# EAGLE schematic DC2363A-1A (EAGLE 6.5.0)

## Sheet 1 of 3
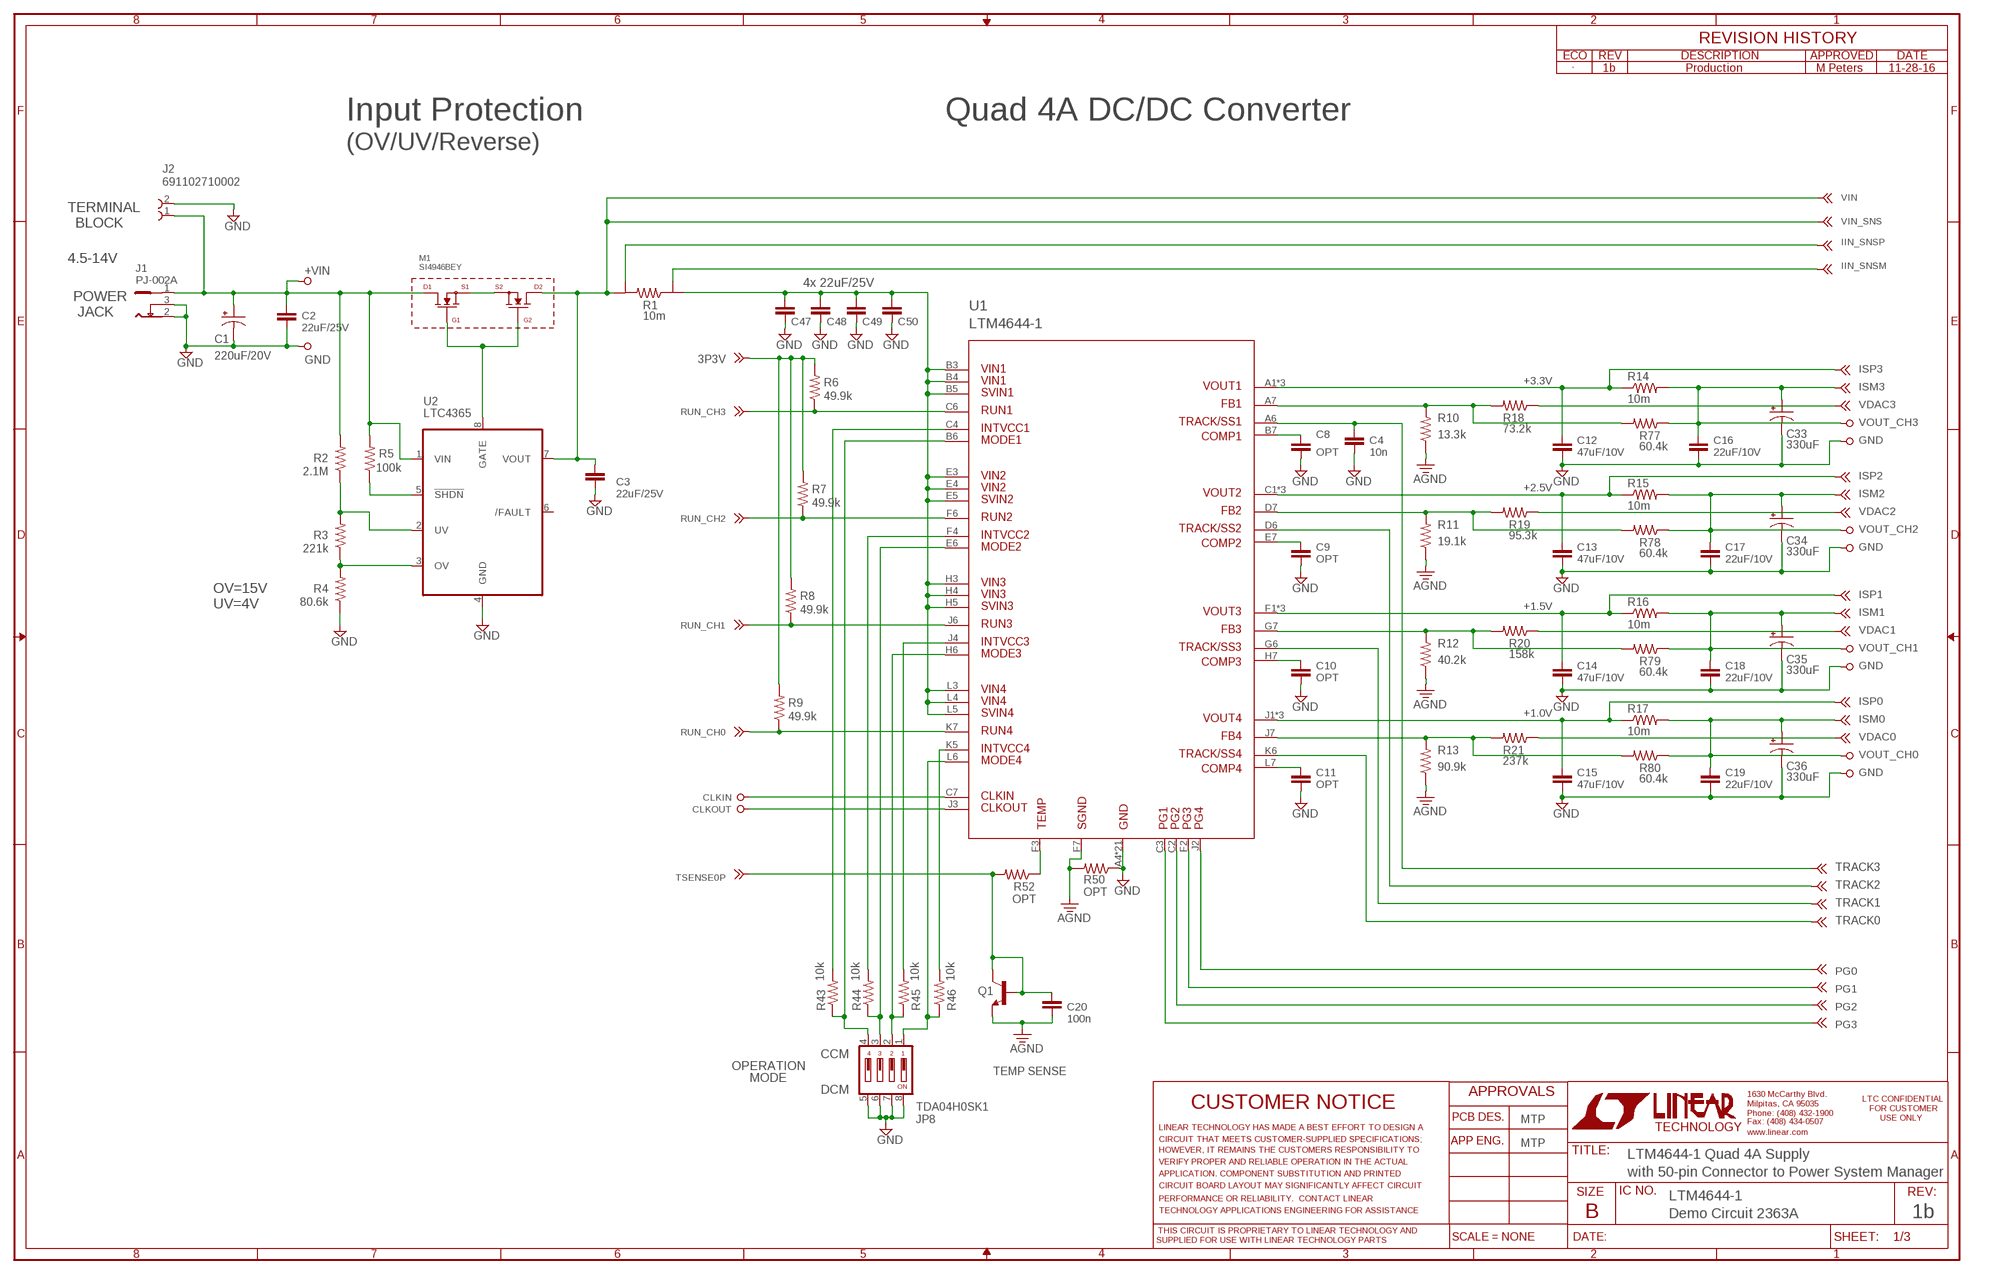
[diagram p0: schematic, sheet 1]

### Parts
C1  220uF/20V  CPOL-USE3.5-8  [E3,5-8]
C2  22uF/25V  CC1210_BOX  [C1210_BOX]
C3  22uF/25V  CC1210_BOX  [C1210_BOX]
C4  10n  CC0603_BOX  [C0603_BOX]
C8  OPT  CC0603_BOX  [C0603_BOX]
C9  OPT  CC0603_BOX  [C0603_BOX]
C10  OPT  CC0603_BOX  [C0603_BOX]
C11  OPT  CC0603_BOX  [C0603_BOX]
C12  47uF/10V  CC1206_BOX  [C1206_BOX]
C13  47uF/10V  CC1206_BOX  [C1206_BOX]
C14  47uF/10V  CC1206_BOX  [C1206_BOX]
C15  47uF/10V  CC1206_BOX  [C1206_BOX]
C16  22uF/10V  CC1210_BOX  [C1210_BOX]
C17  22uF/10V  CC1210_BOX  [C1210_BOX]
C18  22uF/10V  CC1210_BOX  [C1210_BOX]
C19  22uF/10V  CC1210_BOX  [C1210_BOX]
C20  100n  CC0603_BOX  [C0603_BOX]
C33  330uF  CPOL-USD/7343-31R  [D/7343-31R]
C34  330uF  CPOL-USD/7343-31R  [D/7343-31R]
C35  330uF  CPOL-USD/7343-31R  [D/7343-31R]
C36  330uF  CPOL-USD/7343-31R  [D/7343-31R]
C47  22uF/25V  CC1210_BOX  [C1210_BOX]
C48  22uF/25V  CC1210_BOX  [C1210_BOX]
C49  22uF/25V  CC1206_BOX  [C1206_BOX]
C50  22uF/25V  CC1206_BOX  [C1206_BOX]
J1  PJ-002A  [PJ-002A]
J2  691102710002  [691102710002]
JP8  TDA04H0SK1  [SMT_DIP_4]
M1  SI4946BEY  [SOIC-8]
Q1  TEMP SENSE  NPN-SOT23  [SOT-23]
R1  10m  SHUNT  [2512_SHUNT_5MOHM]
R2  2.1M  RR0603_BOX  [R0603_BOX]
R3  221k  RR0603_BOX  [R0603_BOX]
R4  80.6k  RR0603_BOX  [R0603_BOX]
R5  100k  RR0603_BOX  [R0603_BOX]
R6  49.9k  RR0603_BOX  [R0603_BOX]
R7  49.9k  RR0603_BOX  [R0603_BOX]
R8  49.9k  RR0603_BOX  [R0603_BOX]
R9  49.9k  RR0603_BOX  [R0603_BOX]
R10  13.3k  RR0603_BOX  [R0603_BOX]
R11  19.1k  RR0603_BOX  [R0603_BOX]
R12  40.2k  RR0603_BOX  [R0603_BOX]
R13  90.9k  RR0603_BOX  [R0603_BOX]
R14  10m  RR1210_BOX  [R1210_BOX]
R15  10m  RR1210_BOX  [R1210_BOX]
R16  10m  RR1210_BOX  [R1210_BOX]
R17  10m  RR1210_BOX  [R1210_BOX]
R18  73.2k  RR0603_BOX  [R0603_BOX]
R19  95.3k  RR0603_BOX  [R0603_BOX]
R20  158k  RR0603_BOX  [R0603_BOX]
R21  237k  RR0603_BOX  [R0603_BOX]
R43  10k  RR0603_BOX  [R0603_BOX]
R44  10k  RR0603_BOX  [R0603_BOX]
R45  10k  RR0603_BOX  [R0603_BOX]
R46  10k  RR0603_BOX  [R0603_BOX]
R50  OPT  RR0603_BOX  [R0603_BOX]
R52  OPT  RR0603_BOX  [R0603_BOX]
R77  60.4k  RR0603_BOX  [R0603_BOX]
R78  60.4k  RR0603_BOX  [R0603_BOX]
R79  60.4k  RR0603_BOX  [R0603_BOX]
R80  60.4k  RR0603_BOX  [R0603_BOX]
TP1  TURRET_LARGE_2501  [TURRET_LARGE_2501]
TP2  TURRET_LARGE_2501  [TURRET_LARGE_2501]
TP3  TURRET_LARGE_2501  [TURRET_LARGE_2501]
TP4  TURRET_LARGE_2501  [TURRET_LARGE_2501]
TP5  TURRET_LARGE_2501  [TURRET_LARGE_2501]
TP6  TURRET_LARGE_2501  [TURRET_LARGE_2501]
TP7  TURRET_LARGE_2501  [TURRET_LARGE_2501]
TP8  TURRET_LARGE_2501  [TURRET_LARGE_2501]
TP9  TURRET_LARGE_2501  [TURRET_LARGE_2501]
TP10  TURRET_LARGE_2501  [TURRET_LARGE_2501]
TP11  TURRET_SMALL_2308TP  [TURRET_SMALL_2308]
TP12  TURRET_SMALL_2308TP  [TURRET_SMALL_2308]
TP14  TESTPOINT_SMDVIA  [VIA]
TP15  TESTPOINT_SMDVIA  [VIA]
TP16  TESTPOINT_SMDVIA  [VIA]
U1  LTM4644-1  [BGA77_1.27]
U2  LTC4365  [TSOT-23-8]

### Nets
3P3V: R6.2 R7.2 R8.2 R9.2 ; also sheet 3
+VIN: C1.+ C2.1 J1.1 J2.1 M1.7(D1) M1.8(D1) R2.2 R5.2 TP1.TP U2.1(VIN)
AGND: C20.2 Q1.2(E) R10.1 R11.1 R12.1 R13.1 R50.2 U1.F7(SGND)
CLKIN: TP11.TP1 U1.C7(CLKIN)
CLKOUT: TP12.TP1 U1.J3(CLKOUT)
GND: C1.- C2.2 C3.2 C4.2 C8.2 C9.2 C10.2 C11.2 C12.2 C13.2 C14.2 C15.2 C16.2 C17.2 C18.2 C19.2 C33.- C34.- C35.- C36.- C47.2 C48.2 C49.2 C50.2 J1.2 J1.3 J2.2 JP8.5 JP8.6 JP8.7 JP8.8 R4.1 R50.1 TP2.TP TP4.TP TP6.TP TP8.TP TP10.TP U1.A4(GND) U1.A5(GND) U1.B1(GND) U1.B2(GND) U1.C5(GND) U1.D3(GND) U1.D4(GND) U1.D5(GND) U1.E1(GND) U1.E2(GND) U1.F5(GND) U1.G3(GND) U1.G4(GND) U1.G5(GND) U1.H1(GND) U1.H2(GND) U1.J5(GND) U1.K3(GND) U1.K4(GND) U1.L1(GND) U1.L2(GND) U2.4(GND) ; also sheet 2,3
IIN_SNSM: R1.E1 ; also sheet 2
IIN_SNSP: R1.E2 ; also sheet 2
INT1: R43.2 U1.C4(INTVCC1) ; also sheet 2
INT2: R44.2 U1.F4(INTVCC2) ; also sheet 2
INT3: R45.2 U1.J4(INTVCC3) ; also sheet 2
INT4: R46.2 U1.K5(INTVCC4) ; also sheet 2
ISM0: C19.1 C36.+ R17.2 R80.1 TP9.TP ; also sheet 2,3
ISM1: C18.1 C35.+ R16.2 R79.1 TP7.TP ; also sheet 2,3
ISM2: C17.1 C34.+ R15.2 R78.1 TP5.TP ; also sheet 2,3
ISM3: C16.1 C33.+ R14.2 R77.1 TP3.TP ; also sheet 2,3
ISP0: C15.1 R17.1 U1.J1(VOUT4) U1.K1(VOUT4) U1.K2(VOUT4) ; also sheet 2
ISP1: C14.1 R16.1 U1.F1(VOUT3) U1.G1(VOUT3) U1.G2(VOUT3) ; also sheet 2
ISP2: C13.1 R15.1 U1.C1(VOUT2) U1.D1(VOUT2) U1.D2(VOUT2) ; also sheet 2
ISP3: C12.1 R14.1 U1.A1(VOUT1) U1.A2(VOUT1) U1.A3(VOUT1) ; also sheet 2
N$1: M1.2(G1) M1.4(G2) U2.8(GATE)
N$2: M1.1(S1) M1.3(S2)
N$5: R5.1 U2.5(!SHDN)
N$6: R2.1 R3.2 U2.2(UV)
N$7: R3.1 R4.2 U2.3(OV)
N$9: C11.1 U1.L7(COMP4) ; also sheet 3
N$10: C10.1 U1.H7(COMP3) ; also sheet 3
N$11: C9.1 U1.E7(COMP2) ; also sheet 3
N$12: C8.1 U1.B7(COMP1) ; also sheet 3
N$17: R10.2 R18.2 R77.2 U1.A7(FB1) ; also sheet 3
N$18: R11.2 R19.2 R78.2 U1.D7(FB2) ; also sheet 3
N$19: R12.2 R20.2 R79.2 U1.G7(FB3) ; also sheet 3
N$20: R13.2 R21.2 R80.2 U1.J7(FB4) ; also sheet 3
N$42: JP8.1 R46.1 U1.L6(MODE4)
N$43: JP8.2 R45.1 U1.H6(MODE3)
N$52: JP8.3 R44.1 U1.E6(MODE2)
N$53: JP8.4 R43.1 U1.B6(MODE1)
N$58: R52.1 U1.F3(TEMP)
PG0: U1.J2(PG4) ; also sheet 2
PG1: U1.F2(PG3) ; also sheet 2
PG2: U1.C2(PG2) ; also sheet 2
PG3: U1.C3(PG1) ; also sheet 2
RUN_CH0: R9.1 U1.K7(RUN4) ; also sheet 2,3
RUN_CH1: R8.1 U1.J6(RUN3) ; also sheet 2,3
RUN_CH2: R7.1 U1.F6(RUN2) ; also sheet 2,3
RUN_CH3: R6.1 U1.C6(RUN1) ; also sheet 2,3
TRACK0: TP16.1 U1.K6(TRACK4) ; also sheet 3
TRACK1: TP15.1 U1.G6(TRACK3) ; also sheet 3
TRACK2: TP14.1 U1.D6(TRACK2) ; also sheet 3
TRACK3: C4.1 U1.A6(TRACK1) ; also sheet 3
TSENSE0P: C20.1 Q1.1(B) Q1.3(C) R52.2 ; also sheet 2
VDAC0: R21.1 ; also sheet 2
VDAC1: R20.1 ; also sheet 2
VDAC2: R19.1 ; also sheet 2
VDAC3: R18.1 ; also sheet 2
VIN: C3.1 M1.5(D2) M1.6(D2) R1.I2 U2.7(VOUT) ; also sheet 2,3
VIN_U1: C47.1 C48.1 C49.1 C50.1 R1.I1 U1.B3(VIN1) U1.B4(VIN1) U1.B5(SVIN1) U1.E3(VIN2) U1.E4(VIN2) U1.E5(SVIN2) U1.H3(VIN3) U1.H4(VIN3) U1.H5(SVIN3) U1.L3(VIN4) U1.L4(VIN4) U1.L5(SVIN4)
Unconnected: U2.6(/FAULT)

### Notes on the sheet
- 1b | Production | M Peters | 11-28-16
- Input Protection | Quad 4A DC/DC Converter
- (OV/UV/Reverse)
- VIN_SNS
- TERMINAL
    BLOCK
- 4.5-14V
- +VIN
- 4x 22uF/25V
- POWER
   JACK
- GND
- +3.3V
- VOUT_CH3
- +2.5V
- VOUT_CH2
- OV=15V
  UV=4V
- +1.5V
- VOUT_CH1
- +1.0V
- VOUT_CH0
- CCM
- OPERATION
- MODE
- DCM
- MTP
- MTP
- LTM4644-1 Quad 4A Supply
- with 50-pin Connector to Power System Manager
- LTM4644-1
- Demo Circuit 2363A | 1b

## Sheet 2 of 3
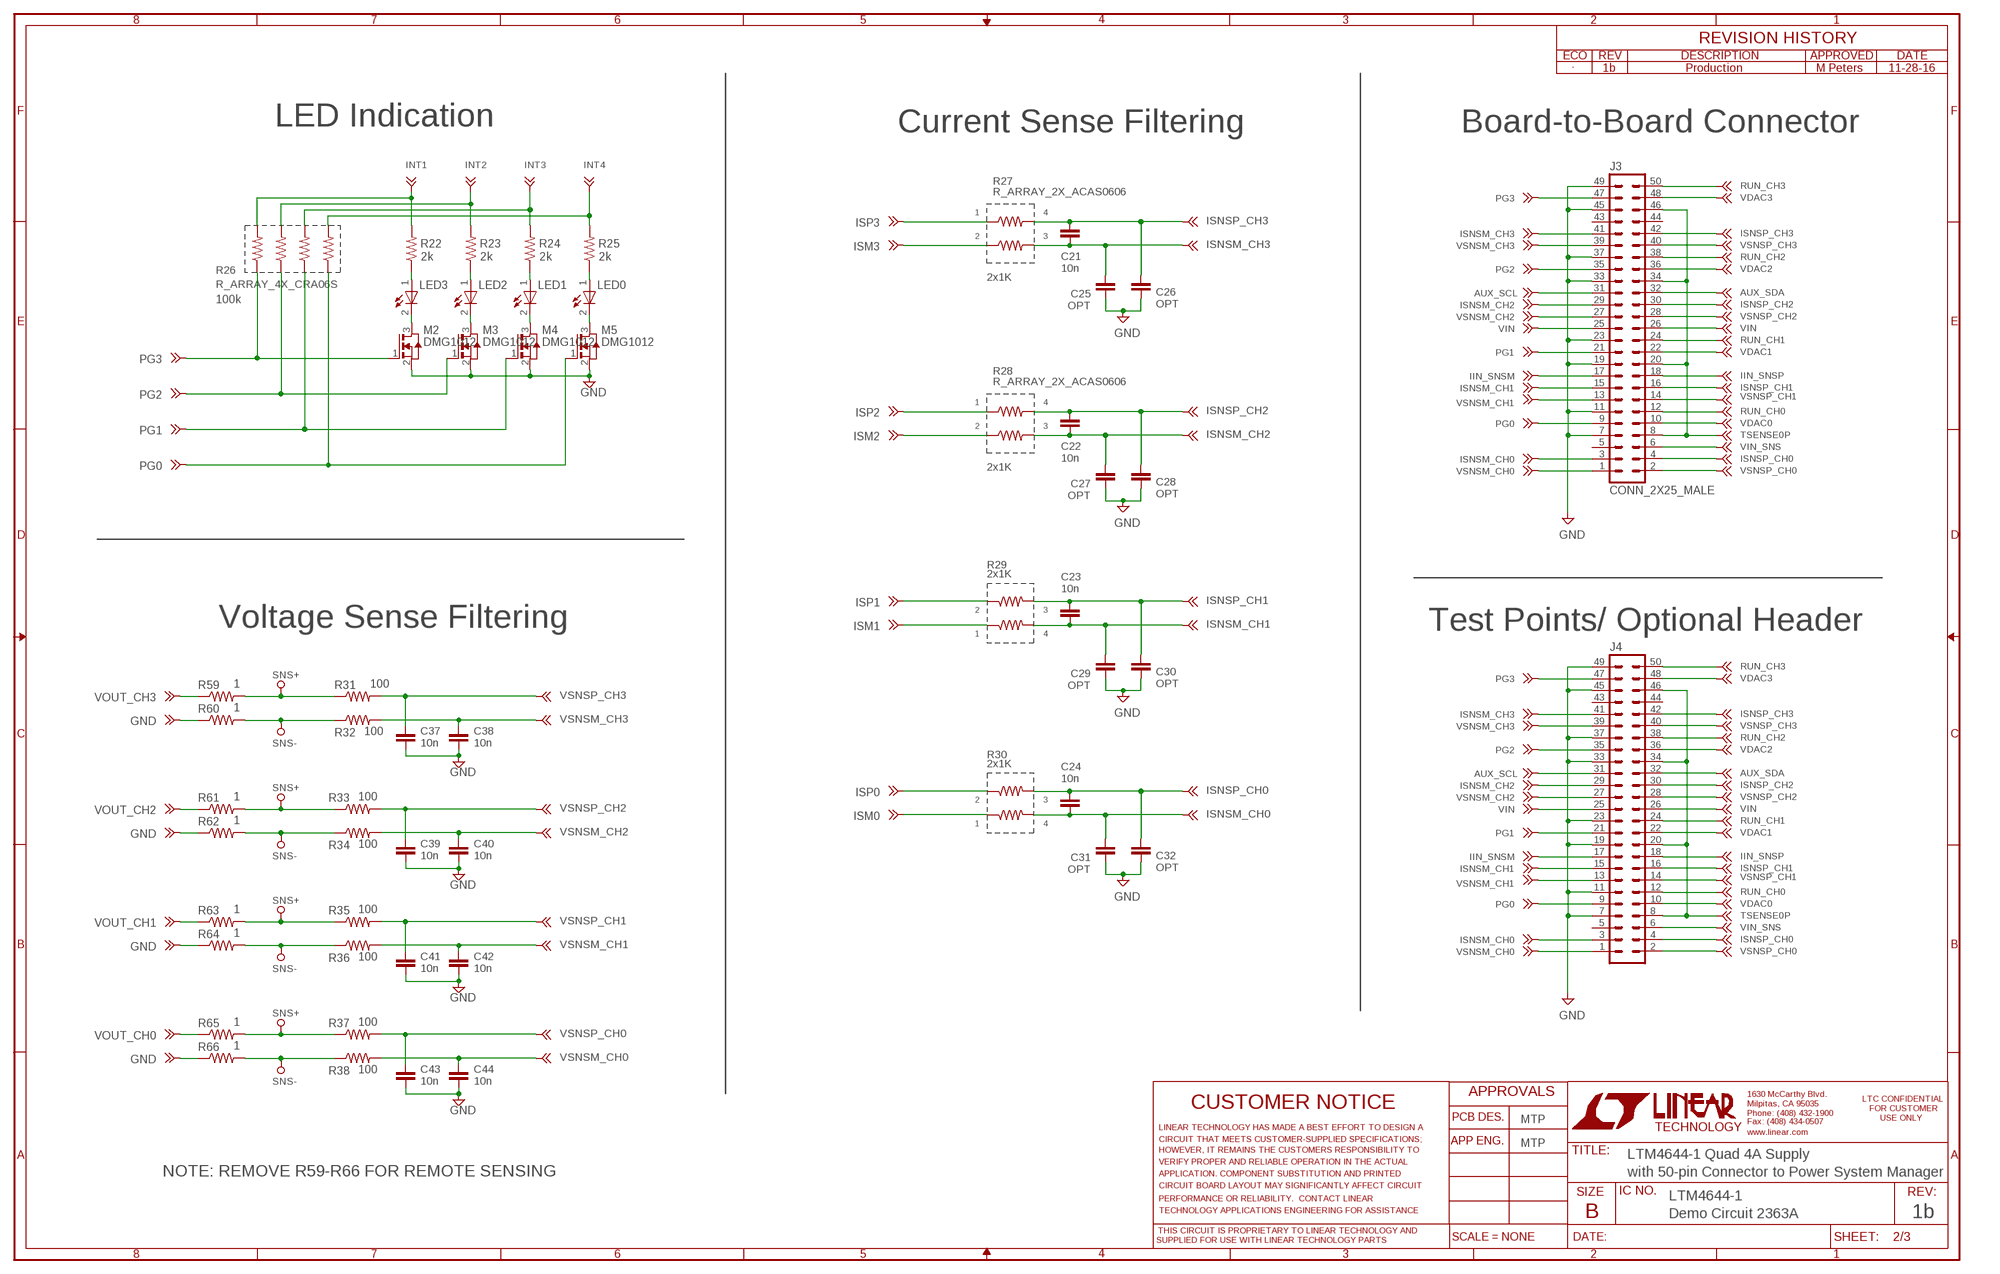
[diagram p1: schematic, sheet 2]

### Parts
C21  10n  CC0603_BOX  [C0603_BOX]
C22  10n  CC0603_BOX  [C0603_BOX]
C23  10n  CC0603_BOX  [C0603_BOX]
C24  10n  CC0603_BOX  [C0603_BOX]
C25  OPT  CC0603_BOX  [C0603_BOX]
C26  OPT  CC0603_BOX  [C0603_BOX]
C27  OPT  CC0603_BOX  [C0603_BOX]
C28  OPT  CC0603_BOX  [C0603_BOX]
C29  OPT  CC0603_BOX  [C0603_BOX]
C30  OPT  CC0603_BOX  [C0603_BOX]
C31  OPT  CC0603_BOX  [C0603_BOX]
C32  OPT  CC0603_BOX  [C0603_BOX]
C37  10n  CC0603_BOX  [C0603_BOX]
C38  10n  CC0603_BOX  [C0603_BOX]
C39  10n  CC0603_BOX  [C0603_BOX]
C40  10n  CC0603_BOX  [C0603_BOX]
C41  10n  CC0603_BOX  [C0603_BOX]
C42  10n  CC0603_BOX  [C0603_BOX]
C43  10n  CC0603_BOX  [C0603_BOX]
C44  10n  CC0603_BOX  [C0603_BOX]
J3  CONN_2X25_MALE  [PINHEAD_2X25_MALE]
J4  CONN_2X25_MALE_NO_SILK  [PINHEAD_2X25_MALE_NO_SILK]
LED0  LED-0603  [CHIPLED_0603]
LED1  LED-0603  [CHIPLED_0603]
LED2  LED-0603  [CHIPLED_0603]
LED3  LED-0603  [CHIPLED_0603]
M2  DMG1012  [SOT-323]
M3  DMG1012  [SOT-323]
M4  DMG1012  [SOT-323]
M5  DMG1012  [SOT-323]
R22  2k  RR0603_BOX  [R0603_BOX]
R23  2k  RR0603_BOX  [R0603_BOX]
R24  2k  RR0603_BOX  [R0603_BOX]
R25  2k  RR0603_BOX  [R0603_BOX]
R26  R_ARRAY_4X_CRA06S  [R_VISHAY_CRA06S]
R27  R_ARRAY_2X_ACAS0606  [R_ARRAY_2X_ACAS]
R28  R_ARRAY_2X_ACAS0606  [R_ARRAY_2X_ACAS]
R29  R_ARRAY_2X_ACAS0606  [R_ARRAY_2X_ACAS]
R30  R_ARRAY_2X_ACAS0606  [R_ARRAY_2X_ACAS]
R31  100  RR0603_BOX  [R0603_BOX]
R32  100  RR0603_BOX  [R0603_BOX]
R33  100  RR0603_BOX  [R0603_BOX]
R34  100  RR0603_BOX  [R0603_BOX]
R35  100  RR0603_BOX  [R0603_BOX]
R36  100  RR0603_BOX  [R0603_BOX]
R37  100  RR0603_BOX  [R0603_BOX]
R38  100  RR0603_BOX  [R0603_BOX]
R59  1  RR0603_BOX  [R0603_BOX]
R60  1  RR0603_BOX  [R0603_BOX]
R61  1  RR0603_BOX  [R0603_BOX]
R62  1  RR0603_BOX  [R0603_BOX]
R63  1  RR0603_BOX  [R0603_BOX]
R64  1  RR0603_BOX  [R0603_BOX]
R65  1  RR0603_BOX  [R0603_BOX]
R66  1  RR0603_BOX  [R0603_BOX]
TP17  TURRET_SMALL_2308TP  [TURRET_SMALL_2308]
TP18  TURRET_SMALL_2308TP  [TURRET_SMALL_2308]
TP19  TURRET_SMALL_2308TP  [TURRET_SMALL_2308]
TP20  TURRET_SMALL_2308TP  [TURRET_SMALL_2308]
TP21  TURRET_SMALL_2308TP  [TURRET_SMALL_2308]
TP22  TURRET_SMALL_2308TP  [TURRET_SMALL_2308]
TP23  TURRET_SMALL_2308TP  [TURRET_SMALL_2308]
TP24  TURRET_SMALL_2308TP  [TURRET_SMALL_2308]

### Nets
AUX_SCL: J3.31 J4.31 ; also sheet 3
AUX_SDA: J3.32 J4.32 ; also sheet 3
GND: C25.1 C26.1 C27.1 C28.1 C29.1 C30.1 C31.1 C32.1 C37.2 C38.2 C39.2 C40.2 C41.2 C42.2 C43.2 C44.2 J3.7 J3.11 J3.19 J3.23 J3.33 J3.37 J3.45 J3.49 J4.7 J4.11 J4.19 J4.23 J4.33 J4.37 J4.45 J4.49 M2.2(S) M3.2(S) M4.2(S) M5.2(S) R60.1 R62.1 R64.1 R66.1 ; also sheet 1,3
IIN_SNSM: J3.17 J4.17 ; also sheet 1
IIN_SNSP: J3.18 J4.18 ; also sheet 1
INT1: R22.2 R26.R1_2 ; also sheet 1
INT2: R23.2 R26.R2_2 ; also sheet 1
INT3: R24.2 R26.R3_2 ; also sheet 1
INT4: R25.2 R26.R4_2 ; also sheet 1
ISM0: R30.P$1 R65.1 ; also sheet 1,3
ISM1: R29.P$1 R63.1 ; also sheet 1,3
ISM2: R28.P$2 R61.1 ; also sheet 1,3
ISM3: R27.P$2 R59.1 ; also sheet 1,3
ISNSM_CH0: C24.2 C31.2 J3.3 J4.3 R30.P$4
ISNSM_CH1: C23.2 C29.2 J3.15 J4.15 R29.P$4
ISNSM_CH2: C22.2 C27.2 J3.29 J4.29 R28.P$3
ISNSM_CH3: C21.2 C25.2 J3.41 J4.41 R27.P$3
ISNSP_CH0: C24.1 C32.2 J3.4 J4.4 R30.P$3
ISNSP_CH1: C23.1 C30.2 J3.16 J4.16 R29.P$3
ISNSP_CH2: C22.1 C28.2 J3.30 J4.30 R28.P$4
ISNSP_CH3: C21.1 C26.2 J3.42 J4.42 R27.P$4
ISP0: R30.P$2 ; also sheet 1
ISP1: R29.P$2 ; also sheet 1
ISP2: R28.P$1 ; also sheet 1
ISP3: R27.P$1 ; also sheet 1
N$27: LED3.P(A) R22.1
N$28: LED2.P(A) R23.1
N$30: LED1.P(A) R24.1
N$31: LED0.P(A) R25.1
N$32: LED3.N(C) M2.3(D)
N$33: LED2.N(C) M3.3(D)
N$34: R31.1 R59.2 TP17.TP1
N$35: R32.1 R60.2 TP18.TP1
N$38: R33.1 R61.2 TP19.TP1
N$39: R34.1 R62.2 TP20.TP1
N$40: LED1.N(C) M4.3(D)
N$41: LED0.N(C) M5.3(D)
N$44: R35.1 R63.2 TP21.TP1
N$45: R36.1 R64.2 TP22.TP1
N$48: R37.1 R65.2 TP23.TP1
N$49: R38.1 R66.2 TP24.TP1
PG0: J3.9 J4.9 M5.1(G) R26.R4_1 ; also sheet 1
PG1: J3.21 J4.21 M4.1(G) R26.R3_1 ; also sheet 1
PG2: J3.35 J4.35 M3.1(G) R26.R2_1 ; also sheet 1
PG3: J3.47 J4.47 M2.1(G) R26.R1_1 ; also sheet 1
RUN_CH0: J3.12 J4.12 ; also sheet 1,3
RUN_CH1: J3.24 J4.24 ; also sheet 1,3
RUN_CH2: J3.38 J4.38 ; also sheet 1,3
RUN_CH3: J3.50 J4.50 ; also sheet 1,3
TSENSE0P: J3.8 J3.20 J3.34 J3.46 J4.8 J4.20 J4.34 J4.46 ; also sheet 1
VDAC0: J3.10 J4.10 ; also sheet 1
VDAC1: J3.22 J4.22 ; also sheet 1
VDAC2: J3.36 J4.36 ; also sheet 1
VDAC3: J3.48 J4.48 ; also sheet 1
VIN: J3.6 J3.25 J3.26 J4.6 J4.25 J4.26 ; also sheet 1,3
VSNSM_CH0: C44.1 J3.1 J4.1 R38.2
VSNSM_CH1: C42.1 J3.13 J4.13 R36.2
VSNSM_CH2: C40.1 J3.27 J4.27 R34.2
VSNSM_CH3: C38.1 J3.39 J4.39 R32.2
VSNSP_CH0: C43.1 J3.2 J4.2 R37.2
VSNSP_CH1: C41.1 J3.14 J4.14 R35.2
VSNSP_CH2: C39.1 J3.28 J4.28 R33.2
VSNSP_CH3: C37.1 J3.40 J4.40 R31.2
Unconnected: J3.5 J3.43 J3.44 J4.5 J4.43 J4.44

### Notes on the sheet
- 1b | Production | M Peters | 11-28-16
- LED Indication | Current Sense Filtering | Board-to-Board Connector
- 2x1K
- 100k
- VIN_SNS
- 2x1K
- 2x1K
- Voltage Sense Filtering | Test Points/ Optional Header
- SNS+
- VOUT_CH3
- SNS-
- 2x1K
- SNS+
- VOUT_CH2
- SNS-
- SNS+
- VOUT_CH1
- VIN_SNS
- SNS-
- SNS+
- VOUT_CH0
- SNS-
- MTP
- MTP
- LTM4644-1 Quad 4A Supply
- NOTE: REMOVE R59-R66 FOR REMOTE SENSING | with 50-pin Connector to Power System Manager
- LTM4644-1
- Demo Circuit 2363A | 1b

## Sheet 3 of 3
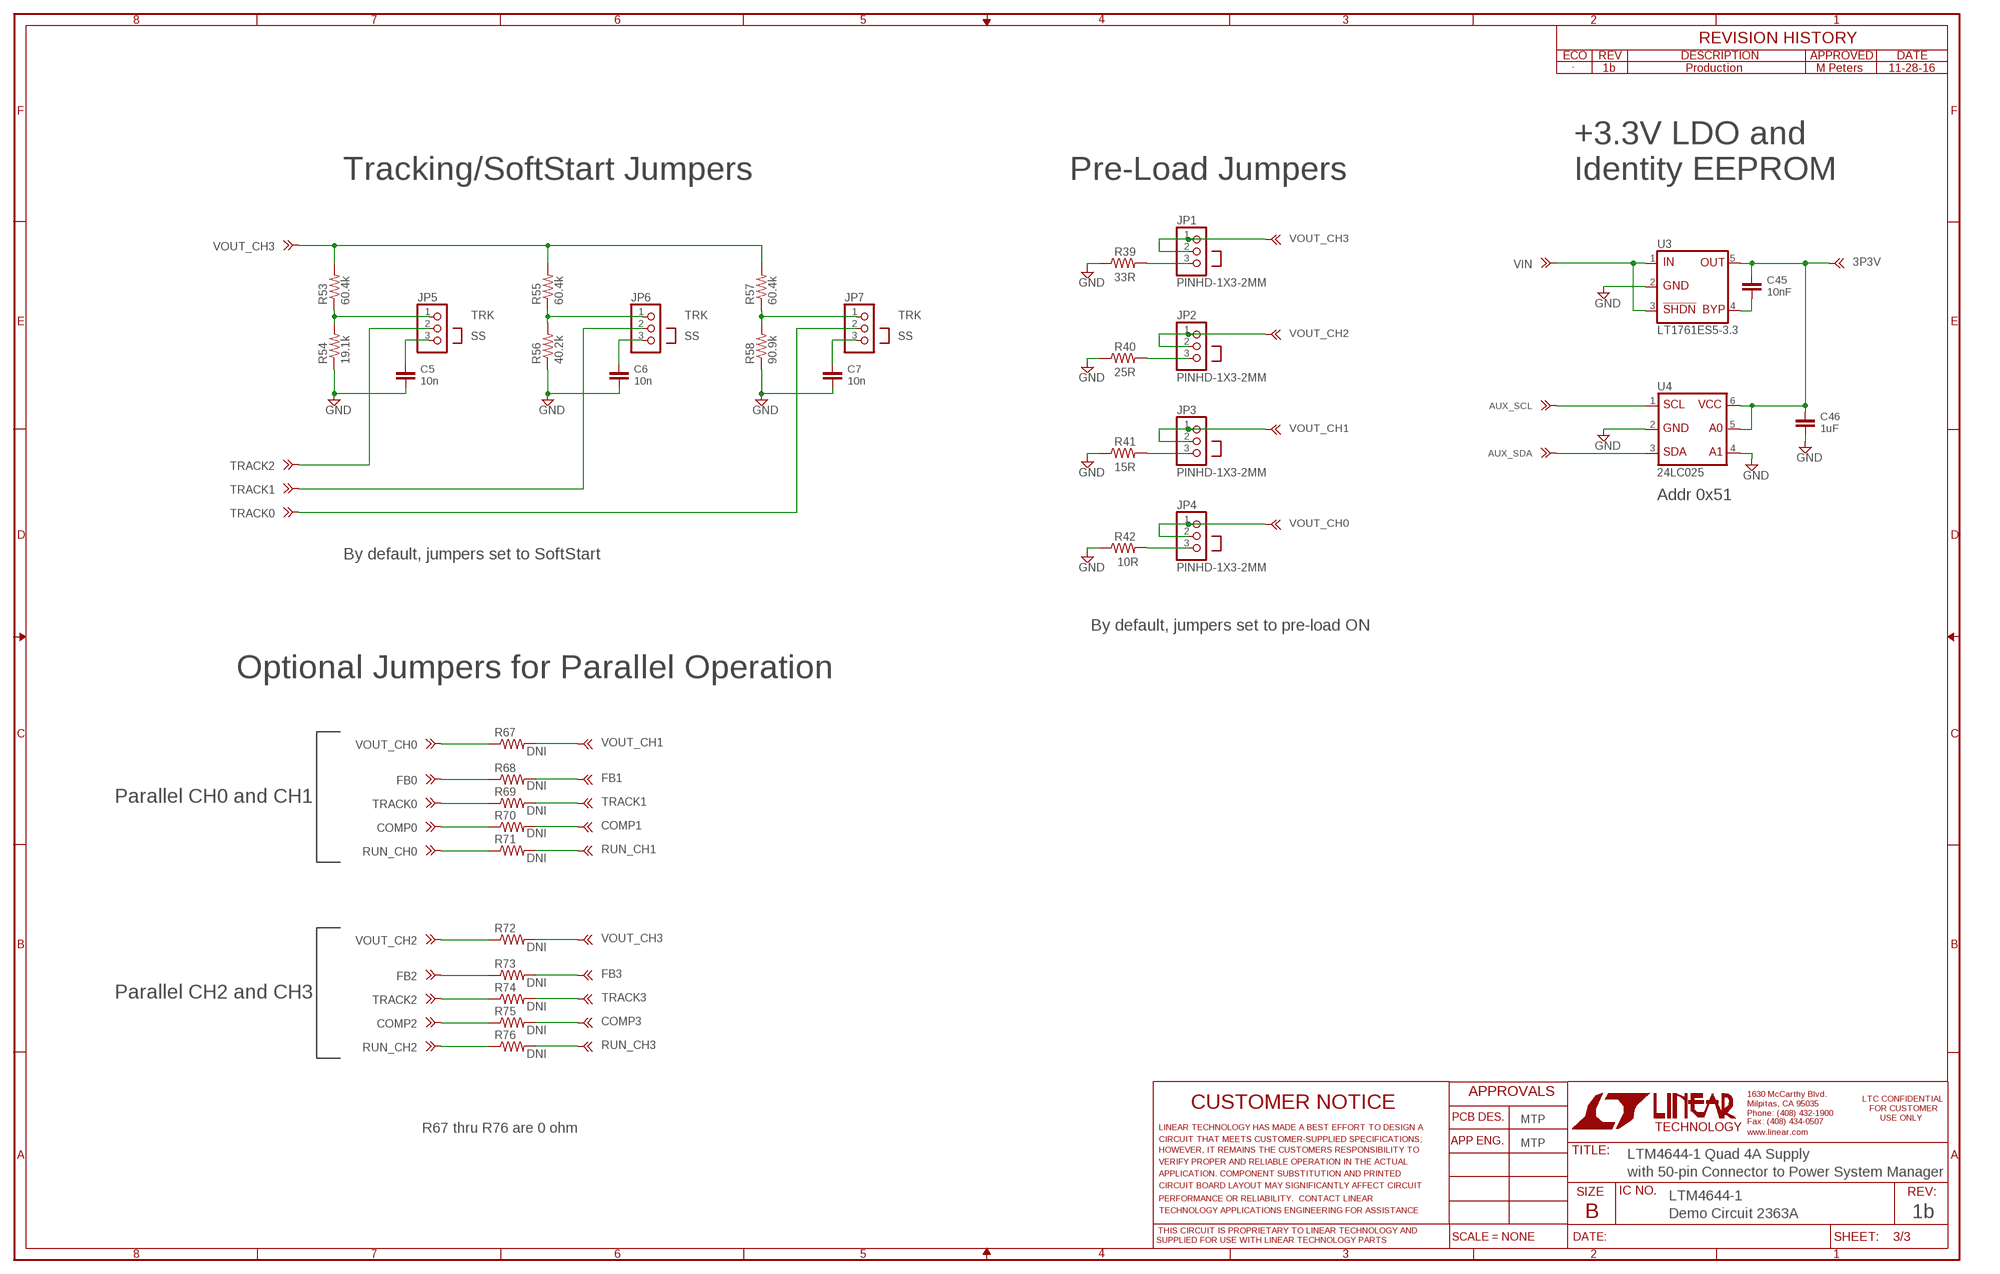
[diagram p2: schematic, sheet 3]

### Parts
C5  10n  CC0603_BOX  [C0603_BOX]
C6  10n  CC0603_BOX  [C0603_BOX]
C7  10n  CC0603_BOX  [C0603_BOX]
C45  10nF  CC0603_BOX  [C0603_BOX]
C46  1uF  CC0603_BOX  [C0603_BOX]
JP1  PINHD-1X3-2MM  [1X03-2MM]
JP2  PINHD-1X3-2MM  [1X03-2MM]
JP3  PINHD-1X3-2MM  [1X03-2MM]
JP4  PINHD-1X3-2MM  [1X03-2MM]
JP5  PINHD-1X3-2MM  [1X03-2MM]
JP6  PINHD-1X3-2MM  [1X03-2MM]
JP7  PINHD-1X3-2MM  [1X03-2MM]
R39  33R  RR1210_BOX  [R1210_BOX]
R40  25R  RR1210_BOX  [R1210_BOX]
R41  15R  RR1210_BOX  [R1210_BOX]
R42  10R  RR1210_BOX  [R1210_BOX]
R53  60.4k  RR0603_BOX  [R0603_BOX]
R54  19.1k  RR0603_BOX  [R0603_BOX]
R55  60.4k  RR0603_BOX  [R0603_BOX]
R56  40.2k  RR0603_BOX  [R0603_BOX]
R57  60.4k  RR0603_BOX  [R0603_BOX]
R58  90.9k  RR0603_BOX  [R0603_BOX]
R67  DNI  R-US_R2010  [R2010]
R68  DNI  RR0603_BOX  [R0603_BOX]
R69  DNI  RR0603_BOX  [R0603_BOX]
R70  DNI  RR0603_BOX  [R0603_BOX]
R71  DNI  RR0603_BOX  [R0603_BOX]
R72  DNI  R-US_R2010  [R2010]
R73  DNI  RR0603_BOX  [R0603_BOX]
R74  DNI  RR0603_BOX  [R0603_BOX]
R75  DNI  RR0603_BOX  [R0603_BOX]
R76  DNI  RR0603_BOX  [R0603_BOX]
U3  LT1761ES5-3.3  LT1761-X  [SOT-23-5]
U4  24LC025  [SOT-23-6]

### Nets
3P3V: C45.1 C46.1 U3.5 U4.5 U4.6 ; also sheet 1
AUX_SCL: U4.1 ; also sheet 2
AUX_SDA: U4.3 ; also sheet 2
GND: C5.2 C6.2 C7.2 C46.2 R39.1 R40.1 R41.1 R42.1 R54.1 R56.1 R58.1 U3.2 U4.2 U4.4 ; also sheet 1,2
ISM0: JP4.1 JP4.2 R67.1 ; also sheet 1,2
ISM1: JP3.1 JP3.2 R67.2 ; also sheet 1,2
ISM2: JP2.1 JP2.2 R72.1 ; also sheet 1,2
ISM3: JP1.1 JP1.2 R53.2 R55.2 R57.2 R72.2 ; also sheet 1,2
N$9: R70.1 ; also sheet 1
N$10: R70.2 ; also sheet 1
N$11: R75.1 ; also sheet 1
N$12: R75.2 ; also sheet 1
N$14: C5.1 JP5.3
N$16: C6.1 JP6.3
N$17: R73.2 ; also sheet 1
N$18: R73.1 ; also sheet 1
N$19: R68.2 ; also sheet 1
N$20: R68.1 ; also sheet 1
N$36: C45.2 U3.4
N$37: C7.1 JP7.3
N$46: JP4.3 R42.2
N$47: JP3.3 R41.2
N$50: JP2.3 R40.2
N$51: JP1.3 R39.2
N$59: JP5.1 R53.1 R54.2
N$60: JP6.1 R55.1 R56.2
N$61: JP7.1 R57.1 R58.2
RUN_CH0: R71.1 ; also sheet 1,2
RUN_CH1: R71.2 ; also sheet 1,2
RUN_CH2: R76.1 ; also sheet 1,2
RUN_CH3: R76.2 ; also sheet 1,2
TRACK0: JP7.2 R69.1 ; also sheet 1
TRACK1: JP6.2 R69.2 ; also sheet 1
TRACK2: JP5.2 R74.1 ; also sheet 1
TRACK3: R74.2 ; also sheet 1
VIN: U3.1 U3.3 ; also sheet 1,2

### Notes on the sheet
- 1b | Production | M Peters | 11-28-16
- +3.3V LDO and
- Tracking/SoftStart Jumpers | Pre-Load Jumpers | Identity EEPROM
- VOUT_CH3 | VOUT_CH3
- TRK | TRK | TRK
- SS | SS | SS | VOUT_CH2
- VOUT_CH1
- Addr 0x51
- VOUT_CH0
- By default, jumpers set to SoftStart
- By default, jumpers set to pre-load ON
- Optional Jumpers for Parallel Operation
- VOUT_CH0
- VOUT_CH1
- FB0
- FB1
- Parallel CH0 and CH1 | TRACK0
- TRACK1
- COMP0
- COMP1
- RUN_CH0
- RUN_CH1
- VOUT_CH2
- VOUT_CH3
- FB2
- FB3
- Parallel CH2 and CH3 | TRACK2
- TRACK3
- COMP2
- COMP3
- RUN_CH2
- RUN_CH3
- MTP
- R67 thru R76 are 0 ohm
- MTP
- LTM4644-1 Quad 4A Supply
- with 50-pin Connector to Power System Manager
- LTM4644-1
- Demo Circuit 2363A | 1b

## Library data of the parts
C1 C33-C36 = rcl:CPOL-US: POLARIZED CAPACITOR, American symbol
C2-C32 C37-C50 = kalin:C: CAPACITOR, European symbol
J1 = kalin:PJ-002A
J2 = Wuerth_Elektronik_eiCan_Terminal_Blocks_Connectors:691102710002: WR-TBL Serie 102 - 5.0mm Horizontal Entry Modular with Pressure Clamp - 1.5mm2 Wires, 2 Pins=>Code : Con_TBL_Screw_PressureClamp_691102710002
J3 = kalin:CONN_2X25_MALE
J4 = kalin:CONN_2X25_MALE_NO_SILK
JP1-JP7 = pinhead:PINHD-1X3-2MM: PIN HEADER
JP8 = kalin:TDA04H0SK1: Ultra-miniature Surface Mount Half-pitch DIP Switch
LED0 LED1-LED3 = kalin:LED-0603: SMD LED in R0603
M1 = kalin:SI4946BEY
M2-M5 = kalin:DMG1012
Q1 = kalin:NPN-SOT23: NPN Transistor SOT23 Package
R1 = kalin:SHUNT: Shunt with Force/Sense
R2-R25 R31-R46 R50 R52-R66 R68-R71 R73-R80 = kalin:R: RESISTOR, American symbol
R26 = kalin:R_ARRAY_4X_CRA06S: Thick Film Resistor Array
R27-R30 = kalin:R_ARRAY_2X_ACAS0606: RESISTOR ARRAY thin film (low TC)
R67 R72 = rcl:R-US_: RESISTOR, American symbol
TP1-TP10 = kalin:TURRET_LARGE_2501: Large Test Turret Mill Max 2501
TP11 TP12 TP17-TP24 = kalin:TURRET_SMALL_2308: Small Test Turret Mill-Max 2308
TP14-TP16 = kalin:TESTPOINT_SMD: Small SMD Test Point
U1 = linear-technology:LTM4644-1: LTM4644-1 Quad 4A DC/DC uModule Regulator (no internal feedback resistor)
U2 = linear-technology:LTC4365
U3 = kalin:LT1761-X: 100mA, Low Noise, LDO Micropower Regulators in TSOT-23
U4 = kalin:24LC025: 2Kbit I2C Serial EEPROM in SOT-23-6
